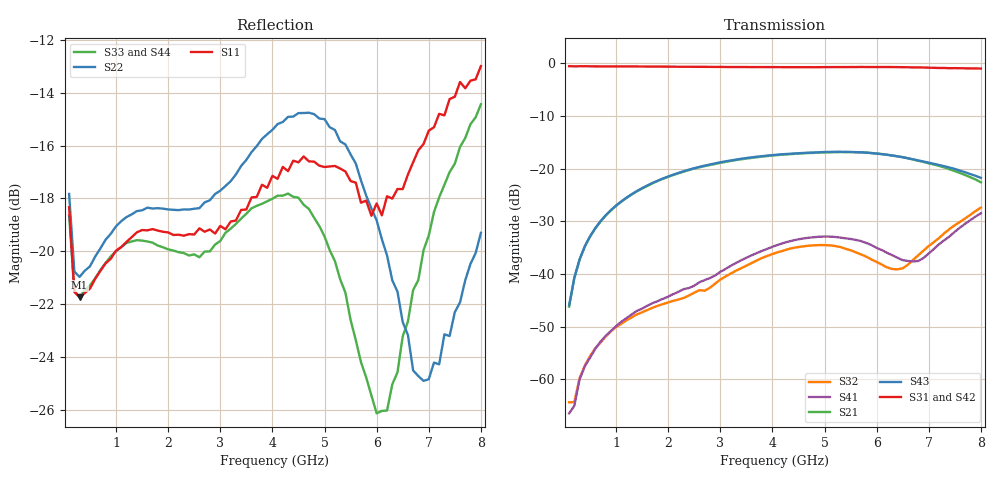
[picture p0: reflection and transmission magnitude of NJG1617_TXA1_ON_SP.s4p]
! Created Wed Nov 12 21:19:33 2008
# hz S ma R 50
! 4 Port Network Data from SP1.SP block
! freq  magS11  angS11  magS12  angS12  magS13  angS13  magS14  angS14
!  magS21  angS21  magS22  angS22  magS23  angS23  magS24  angS24
!  magS31  angS31  magS32  angS32  magS33  angS33  magS34  angS34
!  magS41  angS41  magS42  angS42  magS43  angS43  magS44  angS44
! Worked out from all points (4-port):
!   80 points, 100 MHz to 8 GHz, reference 50 ohm
!   strongest paths, dB at 100 MHz, 2.1 GHz, 4.1 GHz, 6.1 GHz, 8 GHz:
!     S31: -0.6, -0.7, -0.7, -0.7, -1.0
!     S42: -0.5, -0.7, -0.8, -0.7, -0.9
!     S43: -46.0, -21.2, -17.4, -17.3, -21.8
!     S21: -46.2, -21.2, -17.4, -17.2, -22.6
!     S41: -66.5, -43.8, -34.5, -35.5, -28.5
!     S32: -64.4, -45.1, -35.9, -38.2, -27.4
!   lowest |S11| = -21.7 dB at 300 MHz (marker M1), VSWR 1.18, Z = 56.6 + j5.76 ohm
!   |S11| at or under -10 dB: start of sweep to end of sweep
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1e8  0.1212 57.0  0.005092 71.6  0.9389 -7.4  0.001372 -95.7
     0.004891 69.9  0.1284 59.7  0.0007642 -167.6  0.9405 -7.8
     0.9381 -7.2  0.0006026 -67.1  0.1169 58.2  0.004959 77.9
     0.0004741 -60.4  0.9395 -7.7  0.005008 74.1  0.1276 58.0
3e8  0.08178 38.2  0.01361 80.4  0.9363 -6.8  0.001006 -116.4
     0.01357 80.5  0.08941 39.7  0.00105 -130.3  0.9375 -7.0
     0.9356 -6.7  0.001021 -131.6  0.08187 38.2  0.01377 79.7
     0.0009898 -117.1  0.9368 -6.9  0.01368 79.6  0.08467 38.1
1.2e9  0.1042 33.0  0.05261 70.0  0.9325 -19.7  0.003815 176.2
       0.05255 70.1  0.1161 34.5  0.003645 174.4  0.9323 -19.8
       0.9324 -19.6  0.003623 174.5  0.1037 34.2  0.05302 69.9
       0.0038 176.9  0.932 -19.7  0.05291 70.0  0.1041 34.4
3e9  0.1117 9.9  0.1131 43.7  0.9223 -47.4  0.01044 131.2
     0.1131 43.8  0.1303 22.6  0.00882 135.5  0.9202 -47.2
     0.9229 -47.3  0.00882 135.6  0.1046 36.6  0.1147 43.8
     0.01046 131.3  0.9206 -47.1  0.1147 43.9  0.1046 37.1
4.8e9  0.1478 -22.3  0.1412 17.0  0.9174 -76.1  0.02234 68.9
       0.141 17.2  0.1819 -12.3  0.01868 71.2  0.9129 -75.1
       0.9163 -76.0  0.01868 71.3  0.1158 12.2  0.1422 17.3
       0.02229 69.0  0.9122 -75.0  0.1421 17.4  0.1161 13.5
6.2e9  0.1271 -103.8  0.1351 -8.4  0.9208 -101.1  0.01583 -21.0
       0.1351 -8.3  0.09815 -56.3  0.01145 -37.6  0.9223 -99.2
       0.9208 -101.0  0.01151 -37.2  0.04993 67.4  0.1352 -7.0
       0.01585 -20.8  0.9226 -99.1  0.1352 -6.9  0.05303 66.4
8e9  0.2242 169.1  0.07403 -37.3  0.8892 -137.0  0.03768 161.8
     0.07404 -37.3  0.1084 -179.1  0.04255 159.4  0.9028 -133.9
     0.8904 -137.0  0.0425 159.6  0.1899 102.9  0.08158 -29.3
     0.03765 161.8  0.9032 -133.8  0.08159 -29.1  0.1827 104.7
